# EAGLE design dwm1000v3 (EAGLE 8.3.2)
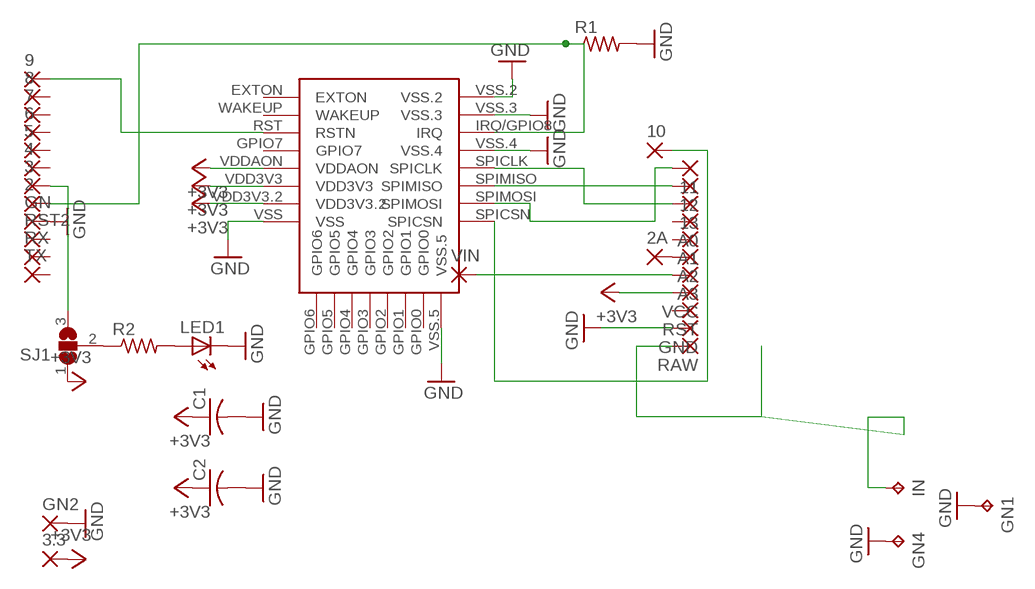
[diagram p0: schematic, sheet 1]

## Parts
2  SMD2  [SMD1,27-2,54]
2A  SMD2  [SMD1,27-2,54]
3  SMD2  [SMD1,27-2,54]
3.3  SMD2  [SMD1,27-2,54]
4  SMD2  [SMD1,27-2,54]
5  SMD2  [SMD1,27-2,54]
6  SMD2  [SMD1,27-2,54]
7  SMD2  [SMD1,27-2,54]
8  SMD2  [SMD1,27-2,54]
9  SMD2  [SMD1,27-2,54]
10  SMD2  [SMD1,27-2,54]
11  SMD2  [SMD1,27-2,54]
12  SMD2  [SMD1,27-2,54]
13  SMD2  [SMD1,27-2,54]
A0  SMD2  [SMD1,27-2,54]
A1  SMD2  [SMD1,27-2,54]
A2  SMD2  [SMD1,27-2,54]
A3  SMD2  [SMD1,27-2,54]
C1  C-USC0805  [C0805]
C2  C-USC0805  [C0805]
GN  SMD2  [SMD1,27-2,54]
GN1  TPTP13SQ  [TP13SQ]
GN2  SMD2  [SMD1,27-2,54]
GN4  TPTP13SQ  [TP13SQ]
GND  SMD2  [SMD1,27-2,54]
IN  TPTP13SQ  [TP13SQ]
LED1  LEDCHIPLED_0805  [CHIPLED_0805]
R1  R-US_R0603  [R0603]
R2  R-US_M0805  [M0805]
RAW  SMD2  [SMD1,27-2,54]
RST  SMD2  [SMD1,27-2,54]
RST2  SMD2  [SMD1,27-2,54]
RX  SMD2  [SMD1,27-2,54]
SJ1  SJ2W  [SJ_2]
TX  SMD2  [SMD1,27-2,54]
U$1  DWM1000  [DWM1000]
VCC  SMD2  [SMD1,27-2,54]
VIN  SMD2  [SMD1,27-2,54]

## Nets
+3V3: 3.3.1(P) C1.1 C2.1 SJ1.1 U$1.VDD3V3 U$1.VDD3V3.2 U$1.VDDAON VCC.1(P)
GND: C1.2 C2.2 GN1.TP GN2.1(P) GN4.TP GN.1(P) GND.1(P) LED1.C R1.2 U$1.VSS U$1.VSS.2 U$1.VSS.3 U$1.VSS.4 U$1.VSS.5
N$1: 10.1(P) U$1.SPICSN
N$2: 9.1(P) U$1.RST(RSTN)
N$3: 12.1(P) U$1.SPIMISO
N$4: 11.1(P) U$1.SPIMOSI
N$5: 13.1(P) U$1.SPICLK
N$6: 2.1(P) R1.1 U$1.IRQ/GPIO8(IRQ)
N$7: LED1.A R2.2
N$8: R2.1 SJ1.2
N$9: 3.1(P) SJ1.3
N$10: IN.TP RAW.1(P)
N$11: A3.1(P) VIN.1(P)
N$13: 2A.1(P) A2.1(P)
Unconnected: 4.1(P) 5.1(P) 6.1(P) 7.1(P) 8.1(P) A0.1(P) A1.1(P) RST2.1(P) RST.1(P) RX.1(P) TX.1(P) U$1.EXTON U$1.GPIO0 U$1.GPIO1 U$1.GPIO2 U$1.GPIO3 U$1.GPIO4 U$1.GPIO5 U$1.GPIO6 U$1.GPIO7 U$1.WAKEUP

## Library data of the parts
2 2A 3 3.3 4-13 A0 A1-A3 GN GN2 GND RAW RST RST2 RX TX VCC VIN = wirepad:SMD2: SMD PAD
C1 C2 = adafruit:C-US: CAPACITOR, American symbol
GN1 GN4 IN = testpad:TP: Test pad
LED1 = adafruit:LED: LED
R1 R2 = adafruit:R-US_: RESISTOR, American symbol
SJ1 = jumper:SJ2W: SMD solder JUMPER
U$1 = dwm1000:DWM1000

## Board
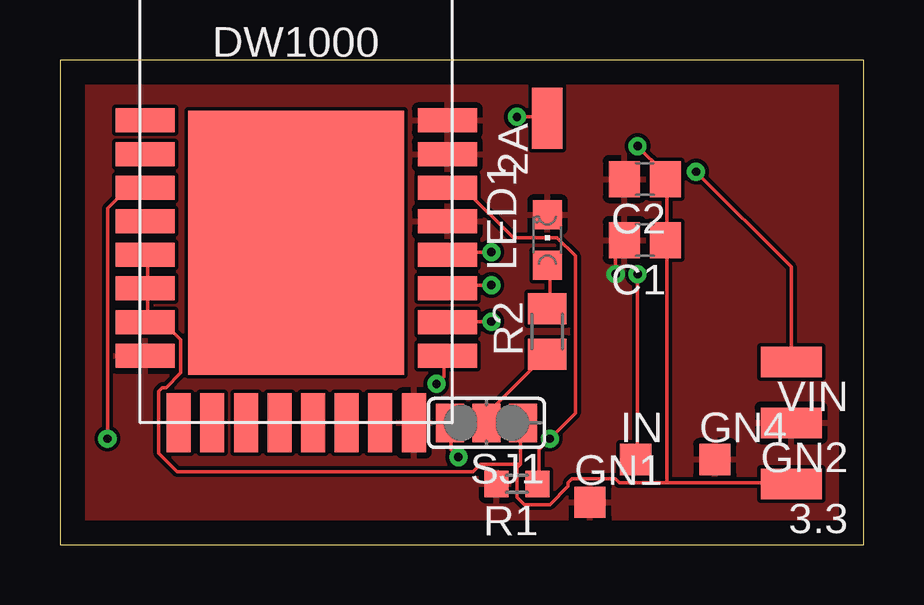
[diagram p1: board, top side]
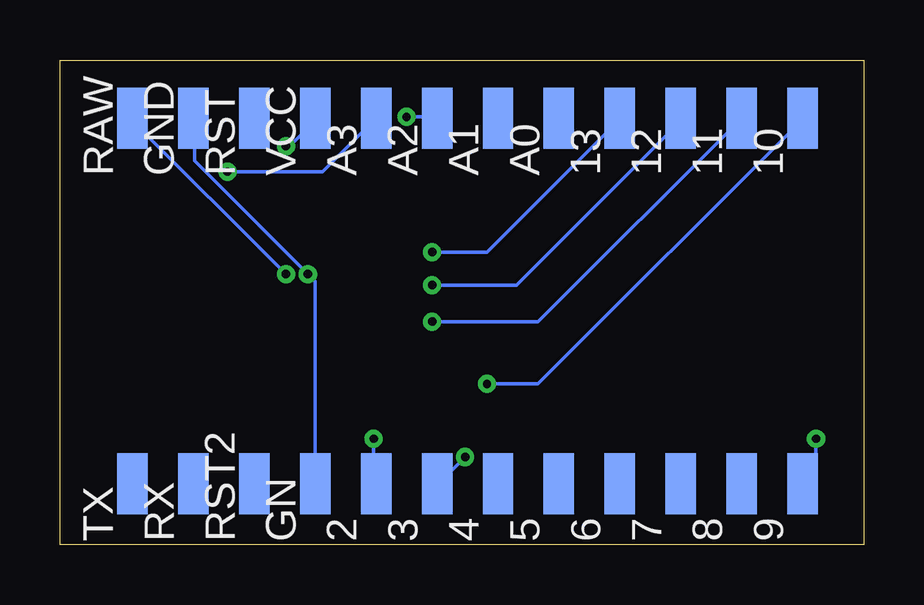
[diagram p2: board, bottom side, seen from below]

Size 33.5 x 20.2 mm. Coordinates in mm from the lower left corner, seen from the top.
Outline: 0,0 33.5,0 33.5,20.2 0,20.2 0,0
Copper layers (1*16): Top 0.035mm / dielectric 1.5mm / Bottom 0.035mm
Design rules "default": minimum track width 6mil, minimum drill 0.35mm, track to track 6mil, track to pad 6mil, pad to pad 6mil, via to via 6mil, smd to smd 6mil, copper to edge 40mil, drill to drill 6mil, minimum pad ring 10mil, minimum via ring 8mil, stop-mask expansion 4mil, vias tented up to drill 0mil, thermal gap 10mil

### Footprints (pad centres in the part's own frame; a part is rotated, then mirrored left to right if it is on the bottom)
SMD1,27-2,54 = smd 1.27 x 2.54: 1 0,0
C0805 = smd 1.3 x 1.5: 1 -0.85,0; 2 0.85,0
TP13SQ = smd 1.3 x 1.3: TP 0,0
CHIPLED_0805 = smd 1.2 x 1.2: A 0,-1.05; C 0,1.05
R0603 = smd 1 x 1.1: 1 -0.85,0; 2 0.85,0
M0805 = smd 1.3 x 1.6: 1 -0.95,0; 2 0.95,0
SJ_2 = smd 1.168 x 1.6: 1 -1.524,0; 2 0,0; 3 1.524,0
DWM1000 = smd 2.45 x 1: EXTON -2.8,12.6; GPIO7 -2.8,8.4; IRQ/GPIO8 9.8,9.8; RST -2.8,9.8; SPICLK 9.8,7; SPICSN 9.8,2.8; SPIMISO 9.8,5.6; SPIMOSI 9.8,4.2; VDD3V3 -2.8,4.2; VDD3V3.2 -2.8,5.6; VDDAON -2.8,7; VSS -2.8,2.8; VSS.2 9.8,12.6; VSS.3 9.8,11.2; VSS.4 9.8,8.4; WAKEUP -2.8,11.2 | smd 9 x 11: GND 3.5,7.5 | smd 1 x 2.45: GPIO0 7,0; GPIO1 5.6,0; GPIO2 4.2,0; GPIO3 2.8,0; GPIO4 1.4,0; GPIO5 0,0; GPIO6 -1.4,0; VSS.5 8.4,0

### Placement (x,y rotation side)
2  20.32,2.54 0 bottom
2A  20.32,17.78 0 top
3  17.78,2.54 0 bottom
3.3  30.48,2.54 90 top
4  15.24,2.54 0 bottom
5  12.7,2.54 0 bottom
6  10.16,2.54 0 bottom
7  7.62,2.54 0 bottom
8  5.08,2.54 0 bottom
9  2.54,2.54 0 bottom
10  2.54,17.78 0 bottom
11  5.08,17.78 0 bottom
12  7.62,17.78 0 bottom
13  10.16,17.78 0 bottom
A0  12.7,17.78 0 bottom
A1  15.24,17.78 0 bottom
A2  17.78,17.78 0 bottom
A3  20.32,17.78 0 bottom
C1  24.38,12.7 180 top
C2  24.38,15.24 180 top
GN  22.86,2.54 0 bottom
GN1  22.1,1.78 0 top
GN2  30.48,5.08 90 top
GN4  27.3,3.56 0 top
GND  27.94,17.78 0 bottom
IN  24,3.56 0 top
LED1  20.32,12.7 0 top
R1  19.05,2.54 180 top
R2  20.32,8.89 90 top
RAW  30.48,17.78 0 bottom
RST  25.4,17.78 0 bottom
RST2  25.4,2.54 0 bottom
RX  27.94,2.54 0 bottom
SJ1  17.78,5.08 180 top
TX  30.48,2.54 0 bottom
U$1  6.35,5.08 0 top
VCC  22.86,17.78 0 bottom
VIN  30.48,7.62 90 top

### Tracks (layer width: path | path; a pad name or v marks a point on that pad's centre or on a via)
+3V3  (via drill 0.35)
  Top 0.152: U$1.VDDAON 3.66,12.04 3.66,10.82 U$1.VDD3V3.2 3.66,10.67 3.66,9.3 U$1.VDD3V3 3.66,9.14 4.42,9.14 5.03,8.53 5.03,7.16 4.42,6.55 4.27,6.55 4.12,6.4 4.12,3.81 4.88,3.05 17.22,3.05 17.53,3.35 19.2,3.35 | 19.2,3.35 19.2,5.03 SJ1.1 | 19.2,3.35 19.05,3.2 19.05,1.98 19.36,1.68 20.42,1.68 21.18,2.44 21.18,2.59 21.34,2.74 23.16,2.74 23.32,2.59 25.3,2.59 | 25.3,2.59 30.48,2.59 3.3.1 | 25.3,2.59 25.3,12.65 C1.1 25.3,12.8 25.3,15.24 C2.1 25.15,15.24 25.15,15.54 v24.08,16.61
  Bottom 0.152: v24.08,16.61 23.93,16.61 22.86,17.68 VCC.1
GND  (via drill 0.35)
  Top 0.152: v23.16,11.28 23.16,12.34 23.47,12.65 C1.2
  Bottom 0.152: GN.1 22.86,10.97 v23.16,11.28 27.89,16 27.89,17.68 GND.1
  pour Top: 0,20.32 35.56,20.32 35.56,-1.27 0,-1.27
N$1  (via drill 0.35)
  Top 0.152: v15.7,6.71 16,7.01 16,7.77 U$1.SPICSN
  Bottom 0.152: v15.7,6.71 13.56,6.71 2.59,17.68 10.1
N$2  (via drill 0.35)
  Top 0.152: v1.98,4.42 1.98,14.02 2.74,14.78 3.5,14.78 U$1.RST
  Bottom 0.152: v1.98,4.42 1.98,3.05 2.44,2.59 9.1
N$3  (via drill 0.35)
  Top 0.152: v17.98,10.82 16.15,10.82 U$1.SPIMISO
  Bottom 0.152: v17.98,10.82 14.48,10.82 7.62,17.68 12.1
N$4  (via drill 0.35)
  Top 0.152: v17.98,9.3 16.15,9.3 U$1.SPIMOSI
  Bottom 0.152: v17.98,9.3 13.56,9.3 11.1
N$5  (via drill 0.35)
  Top 0.152: v17.98,12.19 16.15,12.19 U$1.SPICLK
  Bottom 0.152: v17.98,12.19 15.7,12.19 10.21,17.68 13.1
N$6  (via drill 0.35)
  Top 0.152: R1.1 19.96,2.59 19.96,3.96 v20.42,4.42 21.49,5.49 21.49,12.04 20.73,12.8 18.9,12.8 16.92,14.78 16.15,14.78 U$1.IRQ/GPIO8
  Bottom 0.152: v20.42,4.42 20.42,2.59 2.1
N$7
  Top 0.152: LED1.A 20.42,11.58 20.42,9.91 R2.2
N$8
  Top 0.152: R2.1 20.27,7.92 17.83,5.49 17.83,5.18 SJ1.2
N$9  (via drill 0.35)
  Top 0.152: v16.61,3.66 16.31,3.96 16.31,5.03 SJ1.3
  Bottom 0.152: v16.61,3.66 17.68,2.59 3.1
N$10  (via drill 0.35)
  Top 0.152: v24.08,11.28 24.08,3.66 IN.TP
  Bottom 0.152: v24.08,11.28 30.48,17.68 RAW.1
N$11  (via drill 0.35)
  Top 0.152: VIN.1 30.48,11.58 v26.52,15.54
  Bottom 0.152: v26.52,15.54 22.55,15.54 A3.1
N$13  (via drill 0.35)
  Top 0.152: v19.05,17.83 20.27,17.83 2A.1
  Bottom 0.152: v19.05,17.83 17.83,17.83 A2.1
